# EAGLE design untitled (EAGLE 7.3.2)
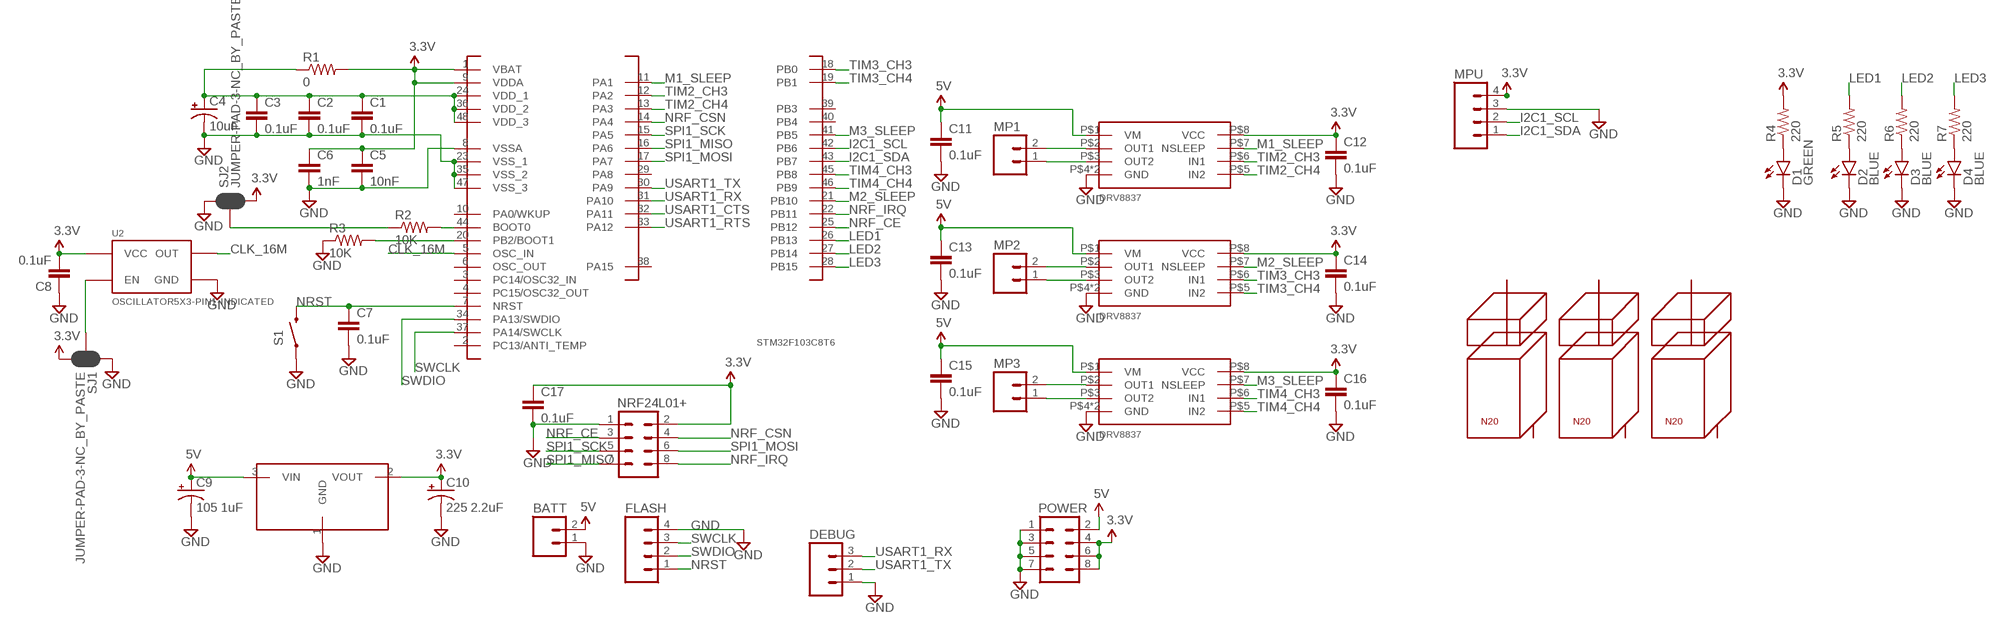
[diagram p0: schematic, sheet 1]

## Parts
BATT  M02JST-PTH-VERT  [JST-2-PTH-VERT]
C1  0.1uF  0.1UF-25V-5%(0603)  [0603-CAP]
C2  0.1uF  0.1UF-25V-5%(0603)  [0603-CAP]
C3  0.1uF  0.1UF-25V-5%(0603)  [0603-CAP]
C4  10uF  10UF-16V-10%(TANT)  [EIA3216]
C5  10nF  10NF/10000PF-50V-10%(0603)  [0603-CAP]
C6  1nF  1NF/1000PF-50V-10%(0603)  [0603-CAP]
C7  0.1uF  0.1UF-25V-5%(0603)  [0603-CAP]
C8  0.1uF  0.1UF-25V-5%(0603)  [0603-CAP]
C9  105 1uF  10UF-16V-10%(TANT)  [EIA3216]
C10  225 2.2uF  10UF-16V-10%(TANT)  [EIA3216]
C11  0.1uF  0.1UF-25V-5%(0603)  [0603-CAP]
C12  0.1uF  0.1UF-25V-5%(0603)  [0603-CAP]
C13  0.1uF  0.1UF-25V-5%(0603)  [0603-CAP]
C14  0.1uF  0.1UF-25V-5%(0603)  [0603-CAP]
C15  0.1uF  0.1UF-25V-5%(0603)  [0603-CAP]
C16  0.1uF  0.1UF-25V-5%(0603)  [0603-CAP]
C17  0.1uF  0.1UF-25V-5%(0603)  [0603-CAP]
D1  GREEN  LED-GREEN0603  [LED-0603]
D2  BLUE  LED-BLUE0603  [LED-0603]
D3  BLUE  LED-BLUE0603  [LED-0603]
D4  BLUE  LED-BLUE0603  [LED-0603]
DEBUG  M03LOCK  [1X03_LOCK]
FLASH  M04LOCK  [1X04_LOCK]
M$1  N20  [N20]
M$2  N20  [N20]
M$3  N20  [N20]
MD1  DRV8837  [PWSON-N8]
MD2  DRV8837  [PWSON-N8]
MD3  DRV8837  [PWSON-N8]
MP1  M02PTH  [1X02]
MP2  M02PTH  [1X02]
MP3  M02PTH  [1X02]
MPU  M04LOCK  [1X04_LOCK]
NRF24L01+  M04X2  [2X4]
POWER  M04X2  [2X4]
R1  0  0OHM-1/10W-5%(0603)  [0603]
R2  10K  10KOHM-1/10W-1%(0603)0603  [0603-RES]
R3  10K  10KOHM-1/10W-1%(0603)0603  [0603-RES]
R4  220  220OHM-1/10W-1%(0603)  [0603-RES]
R5  220  220OHM-1/10W-1%(0603)  [0603-RES]
R6  220  220OHM-1/10W-1%(0603)  [0603-RES]
R7  220  220OHM-1/10W-1%(0603)  [0603-RES]
S1  SWITCH-MOMENTARY-2SMD-REDUNDANT  [TACTILE-SWITCH-SMD]
SJ1  JUMPER-PAD-3-NC_BY_PASTE  [PAD-JUMPER-3-NC_BY_PASTE_YES_SILK_FULL_BOX]
SJ2  JUMPER-PAD-3-NC_BY_PASTE  [PAD-JUMPER-3-NC_BY_PASTE_YES_SILK_FULL_BOX]
U2  OSCILLATOR5X3-PIN1-INDICATED  [CRYSTAL-OSC-SMD-5X3]
U$1  STM32F103C8T6  [LQFP48-7X7]
U$2  AMS1117-3.3  [SOT89]

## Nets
3.3V: C5.1 C6.1 C8.2 C10.A(+) C12.1 C14.1 C16.1 C17.1 MD1.P$8(VCC) MD2.P$8(VCC) MD3.P$8(VCC) MPU.4 NRF24L01+.2 POWER.4 POWER.6 POWER.8 R1.2 R4.2 SJ1.3 SJ2.3 U2.4(VCC) U$1.1(VBAT) U$1.9(VDDA) U$2.2(VOUT)
5V: BATT.2 C9.A(+) C11.1 C13.1 C15.1 MD1.P$1(VM) MD2.P$1(VM) MD3.P$1(VM) POWER.2 U$2.3(VIN)
CLK_16M: U2.3(OUT) U$1.5(OSC_IN)
GND: BATT.1 C1.2 C2.2 C3.2 C4.C(-) C5.2 C6.2 C7.2 C8.1 C9.C(-) C10.C(-) C11.2 C12.2 C13.2 C14.2 C15.2 C16.2 C17.2 D1.C D2.C D3.C D4.C DEBUG.1 FLASH.4 MD1.P$4(GND) MD1.P$9(GND) MD2.P$4(GND) MD2.P$9(GND) MD3.P$4(GND) MD3.P$9(GND) MPU.3 NRF24L01+.1 POWER.1 POWER.3 POWER.5 POWER.7 R3.1 S1.1 S1.2 SJ1.1 SJ2.1 U2.2(GND) U$1.8(VSSA) U$1.23(VSS_1) U$1.35(VSS_2) U$1.47(VSS_3) U$2.1(GND)
I2C1_SCL: MPU.2 U$1.42(PB6)
I2C1_SDA: MPU.1 U$1.43(PB7)
LED1: R5.2 U$1.26(PB13)
LED2: R6.2 U$1.27(PB14)
LED3: R7.2 U$1.28(PB15)
M1_SLEEP: MD1.P$7(NSLEEP) U$1.11(PA1)
M2_SLEEP: MD2.P$7(NSLEEP) U$1.21(PB10)
M3_SLEEP: MD3.P$7(NSLEEP) U$1.41(PB5)
N$1: SJ1.2 U2.1(EN)
N$2: R3.2 U$1.20(PB2/BOOT1)
N$3: R2.1 SJ2.2
N$4: C1.1 C2.1 C3.1 C4.A(+) R1.1 U$1.24(VDD_1) U$1.36(VDD_2) U$1.48(VDD_3)
N$5: R2.2 U$1.44(BOOT0)
N$6: MD1.P$2(OUT1) MP1.2
N$7: MD1.P$3(OUT2) MP1.1
N$11: D1.A R4.1
N$12: D2.A R5.1
N$13: MD2.P$2(OUT1) MP2.2
N$14: MD2.P$3(OUT2) MP2.1
N$15: D3.A R6.1
N$16: D4.A R7.1
N$17: MD3.P$2(OUT1) MP3.2
N$18: MD3.P$3(OUT2) MP3.1
NRF_CE: NRF24L01+.3 U$1.25(PB12)
NRF_CSN: NRF24L01+.4 U$1.14(PA4)
NRF_IRQ: NRF24L01+.8 U$1.22(PB11)
NRST: C7.1 FLASH.1 S1.3 S1.4 U$1.7(NRST)
SPI1_MISO: NRF24L01+.7 U$1.16(PA6)
SPI1_MOSI: NRF24L01+.6 U$1.17(PA7)
SPI1_SCK: NRF24L01+.5 U$1.15(PA5)
SWCLK: FLASH.3 U$1.37(PA14/SWCLK)
SWDIO: FLASH.2 U$1.34(PA13/SWDIO)
TIM2_CH3: MD1.P$6(IN1) U$1.12(PA2)
TIM2_CH4: MD1.P$5(IN2) U$1.13(PA3)
TIM3_CH3: MD2.P$6(IN1) U$1.18(PB0)
TIM3_CH4: MD2.P$5(IN2) U$1.19(PB1)
TIM4_CH3: MD3.P$6(IN1) U$1.45(PB8)
TIM4_CH4: MD3.P$5(IN2) U$1.46(PB9)
USART1_CTS: U$1.32(PA11)
USART1_RTS: U$1.33(PA12)
USART1_RX: DEBUG.3 U$1.31(PA10)
USART1_TX: DEBUG.2 U$1.30(PA9)
Unconnected: U$1.2(PC13/ANTI_TEMP) U$1.3(PC14/OSC32_IN) U$1.4(PC15/OSC32_OUT) U$1.6(OSC_OUT) U$1.10(PA0/WKUP) U$1.29(PA8) U$1.38(PA15) U$1.39(PB3) U$1.40(PB4)

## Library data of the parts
BATT MP1-MP3 = SparkFun-Connectors:M02: Standard 2-pin 0.1" header. Use with
C1-C3 C7 C8 C11-C17 = SparkFun-Capacitors:0.1UF-25V-5%(0603): CAP-08604; PROD_ID: CAP-08604
C4 = SparkFun-Capacitors:10UF-16V-10%(TANT): CAP-00811; PROD_ID: CAP-00811
C5 = SparkFun-Capacitors:10NF/10000PF-50V-10%(0603): CAP-00867; PROD_ID: CAP-00867
C6 = SparkFun-Capacitors:1NF/1000PF-50V-10%(0603): CAP-07886; PROD_ID: CAP-07886
C9 C10 = SparkFun-Capacitors:10UF-16V-10%(TANT): CAP-00811; PROD_ID: CAP-00811; VALUE: 10uF
D1 = SparkFun-LED:LED-GREEN: Various green LEDs; PROD_ID: DIO-00821
D2-D4 = SparkFun-LED:LED-BLUE: Blue LEDs for production use; PROD_ID: DIO-08575
DEBUG = SparkFun-Connectors:M03: Header 3 Standard 3-pin 0.1" header. Use with straight break away headers (SKU : PRT-00116), right angle break away headers (PRT-00553), swiss pins (PRT-00743), machine pins (PRT-00117), and female headers (PRT-00115). Molex polarized connector foot print use with SKU : PRT-08232 with associated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
FLASH MPU = SparkFun-Connectors:M04: Header 4 Standard 4-pin 0.1" header. Use with straight break away headers (SKU : PRT-00116), right angle break away headers (PRT-00553), swiss pins (PRT-00743), machine pins (PRT-00117), and female headers (PRT-00115). Molex polarized connector foot print use with SKU : PRT-08231 with associated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
M$1-M$3 = User-Submitted:N20
MD1-MD3 = User-Submitted:DRV8837
NRF24L01+ POWER = SparkFun-Connectors:M04X2: .1" header, two rows of four.
R1 = SparkFun-Resistors:0OHM-1/10W-5%(0603): RES-08609; PROD_ID: RES-08609
R2 R3 = SparkFun-Resistors:10KOHM-1/10W-1%(0603): RES-00824; PROD_ID: RES-00824
R4-R7 = SparkFun-Resistors:220OHM-1/10W-1%(0603): RES-07861; PROD_ID: RES-07861
S1 = SparkFun-Electromechanical:SWITCH-MOMENTARY-2: Various NO switches- pushbuttons, reed, etc; PROD_ID: SWCH-08247
SJ1 SJ2 = SparkFun-Passives:JUMPER-PAD-3-NC_BY_PASTE
U2 = SparkFun-FreqCtrl:OSCILLATOR: Generic 5x3 and 7x5 oscillators
U$1 = st-microelectronics:STM32F103C8T6
U$2 = User-Submitted:AMS1117-3.3

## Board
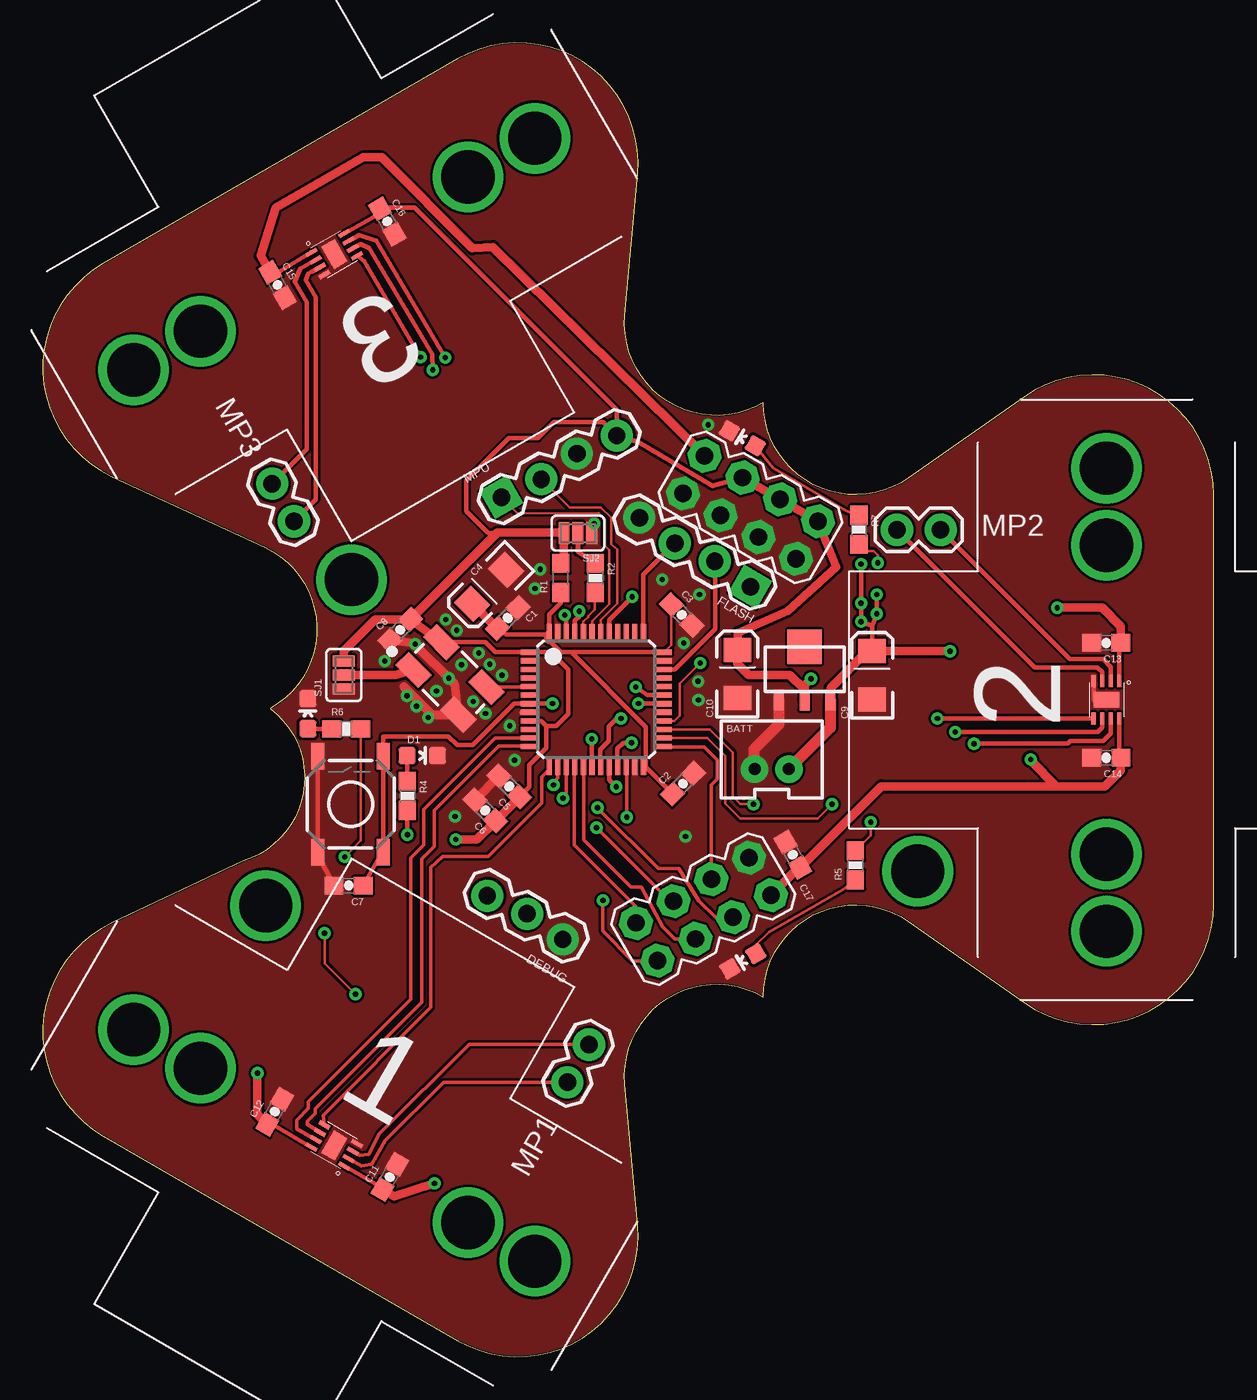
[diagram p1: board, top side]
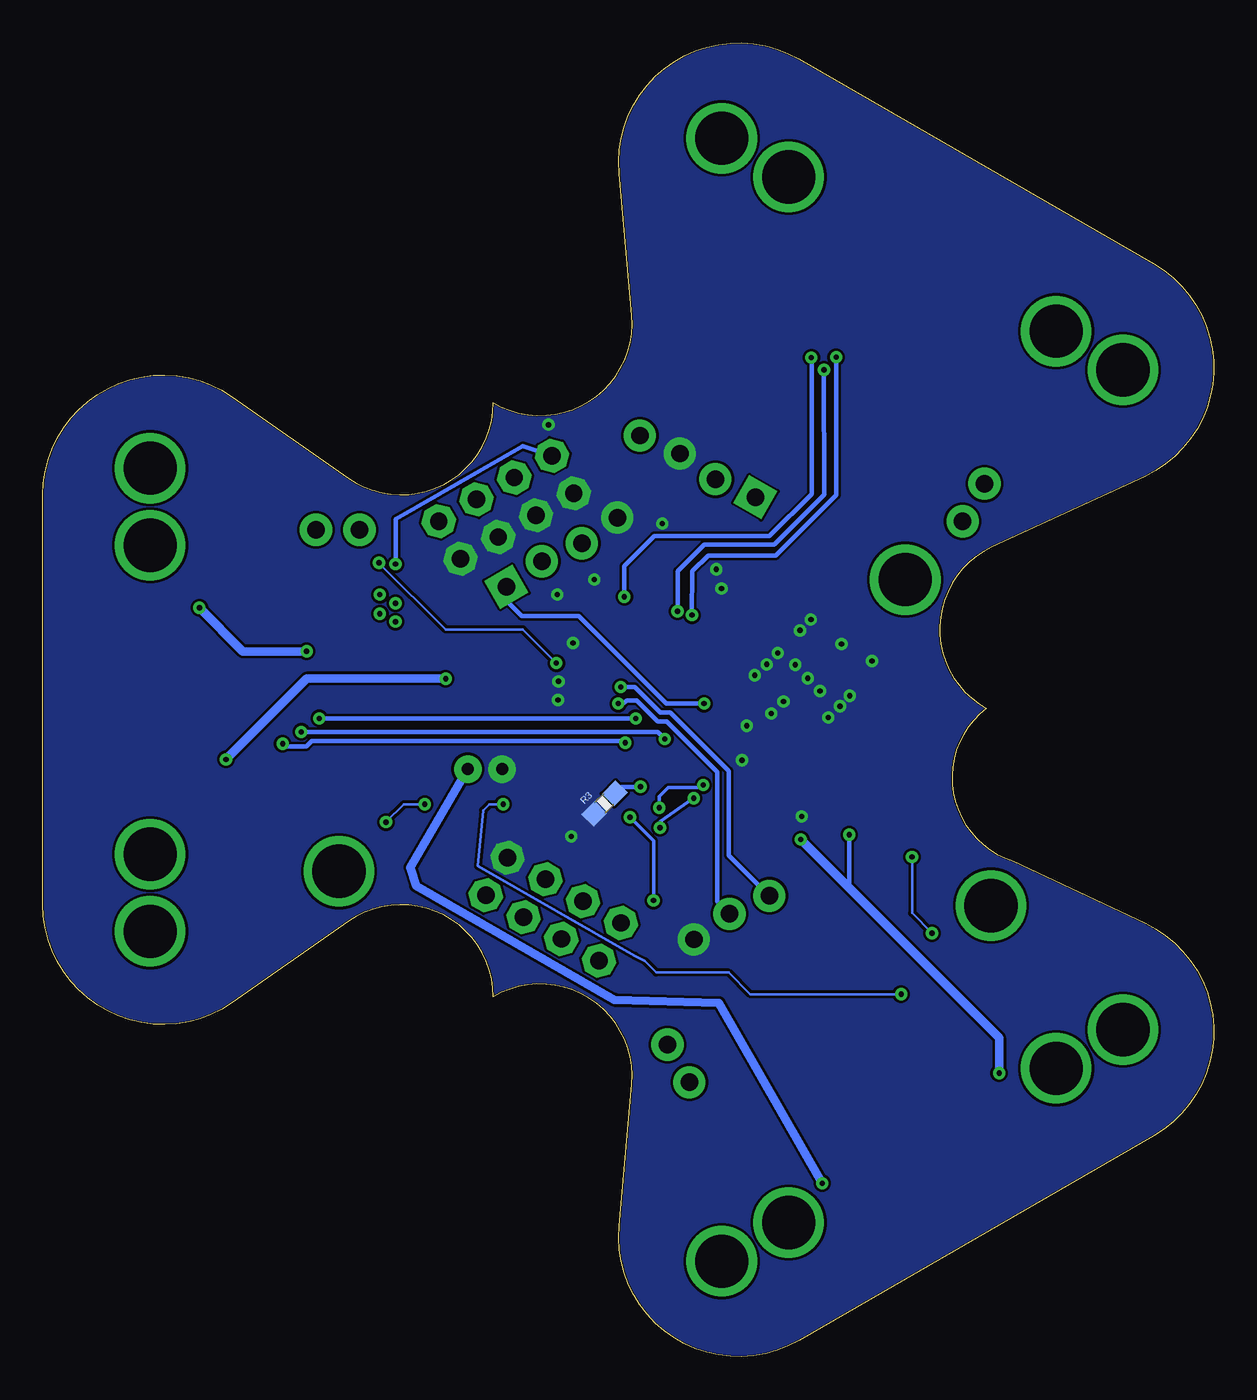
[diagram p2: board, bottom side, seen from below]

Size 68.23 x 76.59 mm. Coordinates in mm from the lower left corner, seen from the top.
Outline: 50.43,25.37 57.22,20.62 arc125 68.23,26.36 68.23,50.23 arc125 57.22,55.96 50.43,51.21 arc-125 41.98,55.61 arc-126 33.91,60.71 34.65,68.96 arc125 24.18,75.65 3.49,63.71 arc125 4,51.32 12.94,47.18 arc-126 13.25,37.79 arc-126 11.67,28.89 4,25.27 arc125 3.49,12.88 24.18,0.93 arc125 34.65,7.62 33.91,15.88 arc-126 41.98,20.97 arc-125 50.43,25.37
Copper layers (1*16): Top 0.035mm / dielectric 1.5mm / Bottom 0.035mm
Design rules "default *": minimum track width 6mil, minimum drill 12mil, track to track 6mil, track to pad 6mil, pad to pad 6mil, via to via 6mil, smd to smd 6mil, copper to edge 3mil, drill to drill 6mil, minimum pad ring 10mil, minimum via ring 8mil, stop-mask expansion 4mil, vias tented up to drill 12mil, thermal gap 10mil

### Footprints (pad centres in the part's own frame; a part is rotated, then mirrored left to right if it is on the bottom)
JST-2-PTH-VERT = drill 0.7 pad 1.6: 1 -1,-0.55; 2 1,-0.55
0603-CAP = smd 1.1 x 1: 1 -0.85,0; 2 0.85,0
EIA3216 = smd 1.4 x 1.6: A 1.4,0; C -1.4,0
LED-0603 = smd 1 x 1: A 0,-0.877; C 0,0.877
1X03_LOCK = drill 1.016 pad 1.88: 1 0,0.127; 2 2.54,-0.127; 3 5.08,0.127
1X04_LOCK = drill 1.016 pad 1.88 square: 1 0,0.127 | drill 1.016 pad 1.88: 2 2.54,-0.127; 3 5.08,0.127; 4 7.62,-0.127
N20 = drill 3.1: P$1 -9,0; P$2 9,0; P$3 -13.5,0; P$4 13.5,0
PWSON-N8 = smd 0.25 x 0.7: P$1 0.75,1.1; P$2 0.25,1.1; P$3 -0.25,1.1; P$4 -0.75,1.1; P$5 -0.75,-1.1; P$6 -0.25,-1.1; P$7 0.25,-1.1; P$8 0.75,-1.1 | smd 1.5 x 0.9: P$9 0,0
1X02 = drill 1.016 pad 1.88: 1 0,0; 2 2.54,0
2X4 = drill 1.016 pad 1.88 octagon: 1 -3.81,-1.27; 2 -3.81,1.27; 3 -1.27,-1.27; 4 -1.27,1.27; 5 1.27,-1.27; 6 1.27,1.27; 7 3.81,-1.27; 8 3.81,1.27
0603 = smd 1.1 x 1: 1 -0.85,0; 2 0.85,0
0603-RES = smd 1.1 x 1: 1 -0.85,0; 2 0.85,0
TACTILE-SWITCH-SMD = smd 1.524 x 0.762: 1 -2.794,1.905; 2 2.794,1.905; 3 -2.794,-1.905; 4 2.794,-1.905
PAD-JUMPER-3-NC_BY_PASTE_YES_SILK_FULL_BOX = smd 0.635 x 1.27: 1 -0.813,0; 2 0,0; 3 0.813,0
CRYSTAL-OSC-SMD-5X3 = smd 1.9 x 1.1: 1 -1.85,-1.15; 2 1.85,-1.15; 3 1.85,1.15; 4 -1.85,1.15
LQFP48-7X7 = smd 0.9 x 0.3: 1 -3.95,2.75; 2 -3.95,2.25; 3 -3.95,1.75; 4 -3.95,1.25; 5 -3.95,0.75; 6 -3.95,0.25; 7 -3.95,-0.25; 8 -3.95,-0.75; 9 -3.95,-1.25; 10 -3.95,-1.75; 11 -3.95,-2.25; 12 -3.95,-2.75; 25 3.95,-2.75; 26 3.95,-2.25; 27 3.95,-1.75; 28 3.95,-1.25; 29 3.95,-0.75; 30 3.95,-0.25; 31 3.95,0.25; 32 3.95,0.75; 33 3.95,1.25; 34 3.95,1.75; 35 3.95,2.25; 36 3.95,2.75 | smd 0.3 x 0.9: 13 -2.75,-3.95; 14 -2.25,-3.95; 15 -1.75,-3.95; 16 -1.25,-3.95; 17 -0.75,-3.95; 18 -0.25,-3.95; 19 0.25,-3.95; 20 0.75,-3.95; 21 1.25,-3.95; 22 1.75,-3.95; 23 2.25,-3.95; 24 2.75,-3.95; 37 2.75,3.95; 38 2.25,3.95; 39 1.75,3.95; 40 1.25,3.95; 41 0.75,3.95; 42 0.25,3.95; 43 -0.25,3.95; 44 -0.75,3.95; 45 -1.25,3.95; 46 -1.75,3.95; 47 -2.25,3.95; 48 -2.75,3.95
SOT89 = smd 0.58 x 1.2: 1 -1.5,-1.8; 2 0,-1.8; 3 1.5,-1.8 | smd 2 x 2: 4 0,1.3

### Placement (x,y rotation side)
BATT  42.47,34.8 0 top
C1  27.09,43.06 45 top
C2  37.3,33.4 45 top
C3  37.23,43.24 315 top
C4  26,44.89 225 top
C5  27.18,33.24 135 top
C6  25.79,31.84 135 top
C7  17.81,27.46 180 top
C8  20.82,42.37 45 top
C9  48.33,39.72 90 top
C10  40.47,39.8 90 top
C11  20.21,10.47 60 top
C12  13.5,14.27 60 top
C13  61.97,41.61 180 top
C14  61.98,34.91 180 top
C15  13.67,62.47 300 top
C16  20.06,66.17 300 top
C17  43.71,29.26 120 top
D1  22.11,35.04 270 top
D2  40.79,23.05 120 top
D3  15.44,37.48 0 top
D4  40.76,53.53 60 top
DEBUG  30.36,24.43 150 top
FLASH  41.29,44.99 150 top
M$1  61.98,38.29 90 top
M$2  16.98,64.27 210 top
M$3  16.98,12.31 330 top
MD1  16.98,12.31 240 top
MD2  61.98,38.29 0 top
MD3  16.98,64.27 120 top
MP1  31.83,18.19 240 top
MP2  49.78,48.19 0 top
MP3  14.63,48.69 120 top
MPU  26.78,49.99 30 top
NRF24L01+  38.49,26.09 210 top
POWER  41.23,49.51 330 top
R1  30.18,45.4 90 top
R2  32.18,45.4 270 top
R3  35.5,32.24 45 bottom
R4  21.23,32.69 270 top
R5  47.35,28.64 90 top
R6  17.68,36.6 0 top
R7  47.56,48.21 270 top
S1  17.93,32.2 90 top
SJ1  17.54,39.73 90 top
SJ2  31.18,48 180 top
U2  23.72,39.53 315 top
U$1  32.25,38.31 0 top
U$2  44.39,40.08 0 top

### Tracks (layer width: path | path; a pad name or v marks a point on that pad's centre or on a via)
3.3V  (via drill 0.3)
  Top 0.203: MD1.P$8 13.62,13.38 C12.1
  Top 0.254: MD2.P$8 62.73,34.91 C14.1 | MD3.P$8 19.31,66.47 C16.1 19.7,66.98 21.67,66.98 33.44,55.21 MPU.4 32.66,54.48 29.78,54.48 28.84,53.54 27.13,53.54 24.67,51.07 24.67,49.3 25.96,48 SJ2.3 | U$1.9 29.05,37.06 29.34,36.77 | 29.34,36.77 29.34,35.48 28.35,34.49 28.35,33.22 C5.1 | U2.4 25.78,41.65 26.37,41.07 U$1.1 29.6,41.06 30.61,40.05 30.61,37.46 29.93,36.77 29.34,36.77 | R4.2 v21.23,30.43 v21.24,30.42
  Top 0.305: SJ2.3 30.37,46.13 R1.2 | MPU.4 34.65,53.34 39.02,50.77 POWER.4
  Top 0.508: POWER.4 POWER.6 POWER.8 46.23,46.02 43.42,43.48 40.49,42.18 C10.A 40.47,40.41 41.13,39.75 43.52,39.75 44.36,38.91 44.36,38.31 U$2.2 44.39,39.14 v44.76,39.52 | C8.2 U2.4 | C8.2 19.36,42.97 17.53,41.14 SJ1.3 | C5.1 C6.1 25.29,30.15 v24.06,30.15 | 30.37,46.13 SJ2.3 30.33,48.03 26.47,48.03 C8.2 | 59.06,33.24 48.85,33.24 C17.1 44.05,28.52 NRF24L01+.2 | 59.06,33.24 61.88,33.24 62.82,34.18 C14.1 | v12.5,16.53 12.5,14.11 C12.1 | v57.56,34.82 57.56,34.74 59.06,33.24
  Bottom 0.254: v21.24,30.42 21.24,27.33 21.04,27.12
  Bottom 0.508: v24.06,30.15 21.04,27.12 12.5,18.59 v12.5,16.53 | v44.76,39.52 52.86,39.52 v57.56,34.82
5V  (via drill 0.3)
  Top 0.203: MD1.P$1 19.36,10.08 C11.1
  Top 0.254: MD2.P$1 62.73,41.61 C13.1 | 48.34,42.59 48.34,41.14 C9.A | MD3.P$1 13.82,63.29 C15.1 | 48.34,42.59 v47.68,42.85 v47.68,43.91 v47.68,46.2 | 48.34,42.59 v48.6,43.3 v48.6,44.42
  Top 0.508: C9.A 48.04,41.12 45.9,38.98 45.9,38.3 U$2.3 | 48.34,41.14 52.84,41.14 v52.86,41.12 | v59.11,43.66 61.73,43.66 62.82,42.57 C13.1 | v22.82,10.1 20.48,9.34 C11.1 | POWER.2 26.22,64.69 25.03,64.61 19.74,69.92 18.68,69.92 13.57,66.98 12.68,64.18 C15.1
  Top 0.635: U$2.3 45.89,36.67 BATT.2
  Bottom 0.254: POWER.2 40.27,53.08 47.66,48.84 47.68,48.81 v47.68,46.2
  Bottom 0.508: v52.86,41.12 56.57,41.12 v59.11,43.66 | BATT.2 46.82,28.52 46.49,27.45 34.93,20.8 28.84,20.62 v22.82,10.1
CLK_16M
  Top 0.203: U$1.5 28.28,39.04 U2.3
GND  (via drill 0.3)
  Top 0.254: MD2.P$4 61.23,38.29 MD2.P$9 | S1.2 S1.1 16.03,29.28 C7.2 | U$1.8 27.87,37.56
  Top 0.508: C8.1 21.57,41.6 24.01,39.21 U2.2 22.69,37.41 21.04,39.06 | C5.2 C6.2
  Top 0.635: U$2.1 42.89,36.86 41.43,35.4 41.43,34.29 BATT.1
  other vias: 23.48,42.97 24.11,42.34 25.41,41.02 26.04,40.36 26.75,39.72 25.08,38.2 25.79,37.49 22.46,37.26 21.77,37.92 21.22,38.53 22.94,38.81 24.39,40.33 21.7,41.55 19.92,40.56 23.65,39.54 27.21,36.77 27.49,34.77 24.01,31.49 38.21,38.27 38.18,39.37 37.35,41.6 38.26,44.42 36.1,45.31 28.68,44.78 28.99,45.89 37.45,30.32 32.14,48.56 38.77,54.33
  pour Top (no thermals): -8.68,-2.19 71.25,-2.19 71.25,77.67 -8.68,77.67
  pour Bottom (no thermals): -3.24,-0.92 76.69,-0.92 76.69,78.94 -3.24,78.94
I2C1_SCL
  Top 0.152: U$1.42 32.5,42.95 33.46,43.91 33.46,47.04 33.13,47.37 33.13,48.92 32.52,49.5 30.7,49.5 MPU.2
I2C1_SDA
  Top 0.152: U$1.43 32,42.89 33,43.89 33,47.01 32.75,47.29 32.75,48.81 32.39,49.17 27.68,49.14 MPU.1
LED1  (via drill 0.3)
  Top 0.152: U$1.26 38.72,36.06 39.76,35.02 39.76,32.25 40.65,31.36 45.14,31.36 v45.98,32.2 | v48.24,31.16 48.24,30.39 R5.2
  Bottom 0.152: v45.98,32.2 47.2,32.2 v48.24,31.16
LED2  (via drill 0.3)
  Top 0.152: R6.2 18.53,30.08 v17.58,29.13 | v16.42,24.68 16.42,22.93 v18.22,21.13 | U$1.27 38.85,36.56 40.19,35.23 40.19,32.69 40.65,32.23 41.38,32.23 v41.41,32.2
  Bottom 0.152: v17.58,29.13 17.58,25.85 v16.42,24.68 | v18.22,21.13 27.01,21.13 28.28,22.4 32.49,22.4 33.15,23.06 33.74,23.36 42.88,28.6 42.58,31.85 42.22,32.2 v41.41,32.2
LED3  (via drill 0.3)
  Top 0.152: U$1.28 36.8,37.06 37.12,37.38 37.12,39.24 v38.31,40.43 | v48.65,46.27 48.65,46.73 48.42,46.96 47.95,46.96 R7.2
  Bottom 0.152: v38.31,40.43 40.27,42.39 44.76,42.39 v48.65,46.27
M1_SLEEP
  Top 0.203: U$1.11 26.35,36.06 22.18,31.9 22.18,29.81 21.44,29.08 21.44,20.82 15.48,14.85 15.48,14.47 14.79,13.79 14.79,13.28 MD1.P$7
M2_SLEEP  (via drill 0.3)
  Top 0.254: MD2.P$7 62.23,36.34 61.78,35.89 59.87,35.89 59.72,35.73 v54.26,35.73 | v34.3,35.78 33.81,35.78 33.48,35.45 33.48,34.38 U$1.21
  Bottom 0.254: v34.3,35.78 34.42,35.89 52.56,35.89 52.89,35.56 54.08,35.56 v54.26,35.73
M3_SLEEP  (via drill 0.3)
  Top 0.254: U$1.41 33,42.95 v34.35,44.29 | v23.45,58.24 19.44,65.07 18.42,65.37 MD3.P$7
  Bottom 0.254: v34.35,44.29 34.35,46.1 32.6,47.85 25.91,47.85 23.43,50.29 23.43,58.21 v23.45,58.24
N$1
  Top 0.508: SJ1.2 20.53,39.75 U2.1
N$2  (via drill 0.3)
  Top 0.254: U$1.20 33,33.63 v33.41,33.22
  Bottom 0.254: v33.41,33.22 34.53,33.22 R3.2
N$3
  Top 0.305: SJ2.2 31.18,46.94 R2.1
N$4
  Top 0.152: C3.1 36.63,41.49 U$1.36
  Top 0.254: U$1.24 35.14,34.36 | 35.14,34.36 C2.1 | U$1.36 30.79,41.06 | 30.79,41.06 30.19,41.06 29.6,41.65 29.45,41.65 29.34,41.75 29.34,42.11 | 29.34,42.11 U$1.48 29.5,43.25 30.18,43.94 R1.1 | 35.14,34.36 35.14,36.72 30.79,41.06 | 29.34,42.11 27.01,42.11 C1.1
  Top 0.508: C1.1 26.44,42.46 C4.A
N$5
  Top 0.152: U$1.44 31.5,42.84 31.78,43.12 31.78,43.18 32.16,43.56 32.16,44.53 R2.2
N$6
  Top 0.203: MD1.P$2 18.55,11.12 19.16,11.2 19.95,12.59 23.35,15.99 MP1.2
N$7
  Top 0.203: MD1.P$3 18.47,11.73 18.98,11.81 19.62,12.97 24.83,18.19 MP1.1
N$8  (via drill 3.1)
  other vias: 17.98,45.29
N$9  (via drill 3.1)
  other vias: 50.98,28.29
N$10  (via drill 3.1)
  other vias: 12.98,26.29
N$11
  Top 0.254: D1.A R4.1
N$12
  Top 0.152: D2.A 41.55,23.99 42.32,24.76 46.64,27.22 R5.1
N$13
  Top 0.254: MD2.P$2 62.23,40.21 61.78,40.66 59.85,40.66 MP2.2
N$14
  Top 0.254: MD2.P$3 61.73,39.9 61.45,40.18 57.8,40.18 MP2.1
N$15
  Top 0.254: D3.A 16.8,36.6 R6.1
N$16
  Top 0.152: D4.A 42.55,51.81 46.84,49.3 R7.1
N$17
  Top 0.254: MD3.P$2 14.99,63.42 14.69,62.66 15.37,61.46 15.37,52.91 MP3.2
N$18
  Top 0.254: MD3.P$3 15.68,63.24 15.48,63.14 15.32,62.76 15.91,61.77 15.91,49.97 MP3.1
NRF_CE
  Top 0.203: NRF24L01+.3 38.95,33.33 39.3,33.68 39.3,34.77 38.54,35.53 36.23,35.53 U$1.25
NRF_CSN  (via drill 0.3)
  Top 0.203: NRF24L01+.4 39.17,25.62 38.23,26.56 37.07,28.47 35.85,28.47 v32.32,32 | v29.75,33.32 29.75,33.47 30,33.73 U$1.14
  Bottom 0.203: v32.32,32 32.32,32.66 31.78,33.19 29.88,33.19 v29.75,33.32
NRF_IRQ  (via drill 0.3)
  Top 0.203: NRF24L01+.8 34.35,23.08 32.62,24.81 32.62,26.56 v32.65,26.59 | v34.02,31.44 34.02,34.35 U$1.22
  Bottom 0.203: v32.65,26.59 32.65,30.07 v34.02,31.44
NRST  (via drill 0.3)
  Top 0.254: 19.84,36.16 23.63,36.16 24.14,35.66 25.05,35.66 27.46,38.07 28,38.07 28,38.06 U$1.7 29.67,38.09 v29.7,38.07 | 19.84,36.16 S1.4 | 19.84,36.16 19.84,30.58 S1.3 19.84,29.52 C7.1
  Bottom 0.254: FLASH.1 41.23,44.09 40.32,43.18 37.01,43.18 31.91,38.07 v29.7,38.07
SPI1_MISO
  Top 0.203: NRF24L01+.7 34.55,26.23 30.97,29.81 30.97,34.33 U$1.16
SPI1_MOSI
  Top 0.203: NRF24L01+.6 36.81,24.35 36.13,25.04 34.86,27.38 34.27,27.38 31.53,30.12 31.53,34.34 U$1.17
SPI1_SCK  (via drill 0.3)
  Top 0.203: NRF24L01+.5 36.54,26.55 v32.26,30.83 | v30.31,32.56 30.51,32.89 30.51,34.35 U$1.15
  Bottom 0.203: v32.26,30.83 32.26,31.19 v30.31,32.56
SWCLK
  Top 0.254: U$1.37 35,45.59 FLASH.3
SWDIO
  Top 0.254: U$1.34 36.82,40.06 39.17,42.41 39.17,46.35 FLASH.2
TIM2_CH3
  Top 0.203: U$1.12 28.35,35.61 26.58,35.61 22.82,31.85 22.82,29.74 22.08,29 22.08,20.65 15.88,14.45 15.88,14.19 15.4,13.71 15.4,13.53 MD1.P$6
TIM2_CH4
  Top 0.203: U$1.13 29.5,34.24 29.06,33.8 29.06,32.28 25.94,29.15 23.3,29.15 22.61,28.52 22.61,20.37 16.35,14.05 MD1.P$5
TIM3_CH3  (via drill 0.3)
  Top 0.254: MD2.P$6 61.73,36.67 61.47,36.42 v53.17,36.42 | v31.99,36.01 31.99,34.38 U$1.18
  Bottom 0.254: v53.17,36.42 32.39,36.42 v31.99,36.01
TIM3_CH4  (via drill 0.3)
  Top 0.254: MD2.P$5 v52.14,37.19 v52.13,37.21 | v33.69,37.21 33.43,37.21 32.98,36.75 32.98,35.89 32.49,35.4 U$1.19
  Bottom 0.254: v52.13,37.21 v33.69,37.21
TIM4_CH3  (via drill 0.3)
  Top 0.254: U$1.45 31,42.9 31.25,43.15 v31.25,43.45 | MD3.P$6 18.52,64.84 19.01,64.61 22.69,58.44 v22.71,57.53
  Bottom 0.254: v31.25,43.45 31.25,45.79 29.7,47.34 25.61,47.34 22.69,50.26 v22.71,57.53
TIM4_CH4  (via drill 0.3)
  Top 0.254: U$1.46 30.5,43.04 v30.41,43.23 | v22,58.26 18.73,63.85 MD3.P$5
  Bottom 0.254: v30.41,43.23 30.39,45.79 29.47,46.71 25.53,46.71 22,50.24 v22,58.26
USART1_RX  (via drill 0.3)
  Top 0.254: U$1.31 35.23,38.56 v34.55,39.04
  Bottom 0.254: v34.55,39.04 33.74,39.04 32.26,37.56 31.68,37.56 28.25,34.13 28.25,29.21 DEBUG.3
USART1_TX  (via drill 0.3)
  Top 0.254: U$1.30 v34.71,38.06 v34.7,38.07
  Bottom 0.254: v34.7,38.07 34.4,38.07 34.22,38.25 33.61,38.25 32.39,37.03 31.88,37.03 28.94,34.08 28.94,26.52 DEBUG.2

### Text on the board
tNames: 3 | 2 | 1

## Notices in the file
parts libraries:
SparkFun-Capacitors: Licensing: Creative Commons ShareAlike 4.0 International - https://creativecommons.org/licenses/by-sa/4.0
